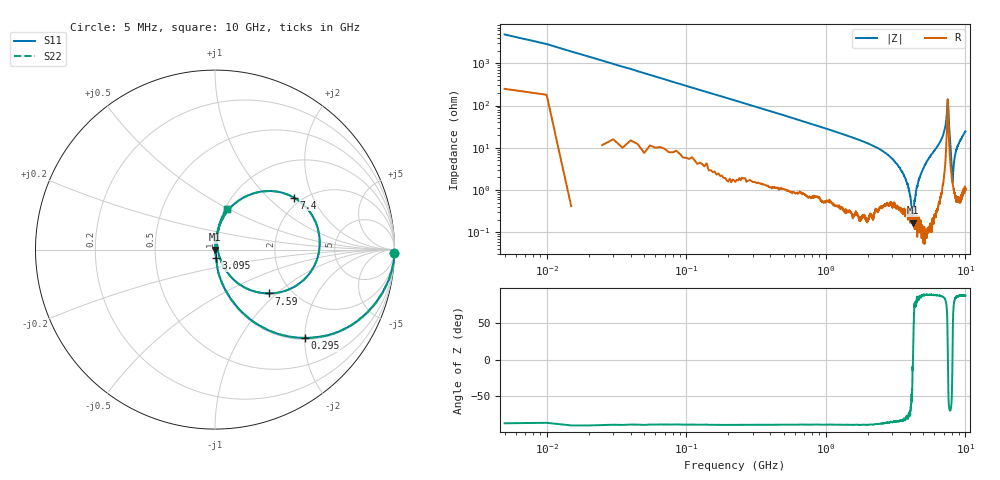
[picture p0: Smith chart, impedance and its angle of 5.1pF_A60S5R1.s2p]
! Amotech Co.,Ltd.
! http://www.amotech.co.kr/
! Part Number: A60S5R1
! These Parameters are Measured in Series Mode Connection
! Operation Temp=25[degC], DC Bias Voltage=0[V]
! Freq. Start=5[MHz] Stop=10[GHz], 2000[Steps]
! Date: Monday, July 13, 2020, 01:29:13
# GHZ S RI R 50.000000
!Freq.(Hz) S11(Real) S11(Imag) S21(Real) S21(Imag) S12(Real) S12(Imag) S22(Real) S22(Imag)
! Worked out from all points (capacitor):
!   2000 points, 5 MHz to 10 GHz, reference 50 ohm
!   read as one part in series: C = 5.45 pF near 55 MHz
!   lowest |Z| = 167 mohm at 4.195 GHz (marker M1)
!   series resonance near 4.208 GHz, so ESL is about 260 pH
!   S11 on the Smith chart (normalised r, x): 5 MHz: 6, -96; 295 MHz: 1.03, -2.00; 3.095 GHz: 1.01, -0.10; 7.4 GHz: 1.81, +1.45; 7.59 GHz: 1.55, -0.89; 10 GHz: 1.02, +0.49
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0.005  0.9985 -0.0207  0.0015 0.0207  0.0015 0.0207  0.9985 -0.0207
0.065  0.9489 -0.2089  0.0511 0.2089  0.0511 0.2089  0.9489 -0.2089
0.105  0.8807 -0.3145  0.1193 0.3145  0.1193 0.3145  0.8807 -0.3145
0.295  0.4991 -0.4919  0.5009 0.4919  0.5009 0.4919  0.4991 -0.4919
0.73  0.1415 -0.3395  0.8585 0.3395  0.8585 0.3395  0.1415 -0.3395
1.675  0.0276 -0.1551  0.9724 0.1551  0.9724 0.1551  0.0276 -0.1551
3.095  0.00694 -0.0479  0.9931 0.0479  0.9931 0.0479  0.00694 -0.0479
3.34  0.00493 -0.0346  0.9951 0.0346  0.9951 0.0346  0.00493 -0.0346
3.9  0.00235 -0.0115  0.9977 0.0115  0.9977 0.0115  0.00235 -0.0115
4.195  0.00162 -0.00042  0.9984 0.00042  0.9984 0.00042  0.00162 -0.00042
4.47  0.00216 0.0112  0.9978 -0.0112  0.9978 -0.0112  0.00216 0.0112
5.005  0.00166 0.033  0.9983 -0.033  0.9983 -0.033  0.00166 0.033
6.67  0.0283 0.1432  0.9717 -0.1432  0.9717 -0.1432  0.0283 0.1432
7.175  0.1191 0.2635  0.8809 -0.2635  0.8809 -0.2635  0.1191 0.2635
7.4  0.4389 0.2902  0.5611 -0.2902  0.5611 -0.2902  0.4389 0.2902
7.49  0.5777 -0.0205  0.4223 0.0205  0.4223 0.0205  0.5777 -0.0205
7.59  0.3021 -0.2441  0.6979 0.2441  0.6979 0.2441  0.3021 -0.2441
7.745  0.0786 -0.1402  0.9214 0.1402  0.9214 0.1402  0.0786 -0.1402
8.07  0.0158 -0.000479  0.9842 0.000479  0.9842 0.000479  0.0158 -0.000479
8.335  0.0109 0.0506  0.9891 -0.0506  0.9891 -0.0506  0.0109 0.0506
8.785  0.0175 0.1063  0.9825 -0.1063  0.9825 -0.1063  0.0175 0.1063
10  0.0661 0.2285  0.9339 -0.2285  0.9339 -0.2285  0.0661 0.2285
